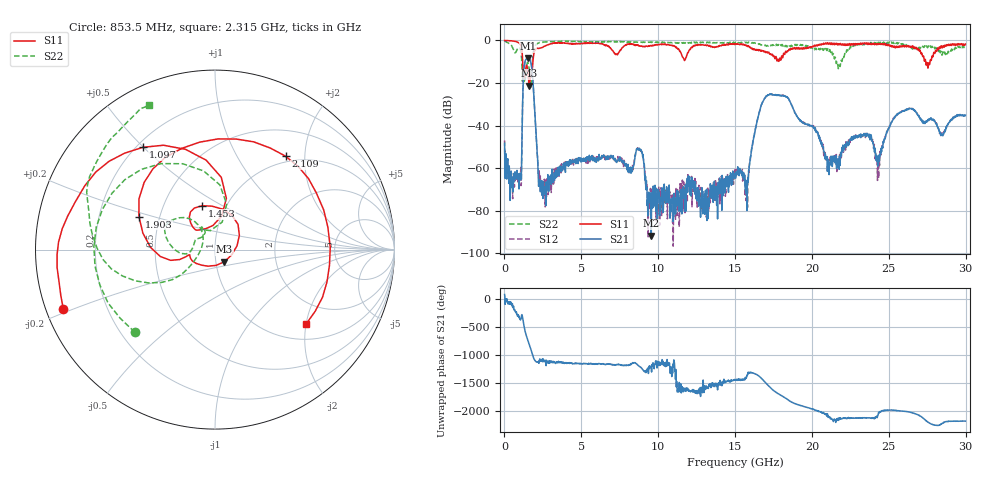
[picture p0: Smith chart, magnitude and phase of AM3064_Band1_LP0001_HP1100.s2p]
# Hz S DB R 50.0
!freq dBS11 angS11 dBS21 angS21 dBS12 angS12 dBS22 angS22
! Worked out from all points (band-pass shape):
!   1600 points, 10 MHz to 29.98 GHz, reference 50 ohm
!   highest |S21| = -8.39 dB at 1.528 GHz (marker M1); lowest = -91.7 dB at 9.551 GHz (marker M2)
!   |S21| within 3 dB of the highest: 1.301 GHz to 1.745 GHz (443.5 MHz wide, 29.1 % of centre)
!   lowest |S11| = -21.4 dB at 1.603 GHz (marker M3), VSWR 1.19, Z = 55 - j7.47 ohm
!   |S11| at or under -10 dB: 1.186 GHz to 1.85 GHz (664 MHz wide, 43.7 % of centre); 27.4 GHz to 27.68 GHz (283.1 MHz wide, 1.03 % of centre)
!   |S22| runs from -22.4 to -0.2 dB; largest |S21 - S12| = 0.0049
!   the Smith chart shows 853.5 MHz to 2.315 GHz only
!   S11 on the Smith chart (normalised r, x): 853.5 MHz: 0.05, -0.19; 1.097 GHz: 0.22, +0.50; 1.453 GHz: 0.77, +0.40; 1.903 GHz: 0.38, +0.18; 2.109 GHz: 0.90, +1.63; 2.315 GHz: 1.36, -2.00
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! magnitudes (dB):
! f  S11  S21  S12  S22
! 10 MHz  -0.1  -48.4  -46.9  -0.2
! 853.5 MHz  -0.8  -64.2  -63.4  -3.9
! 1.097 GHz  -3.1  -65.2  -67.3  -7.1
! 1.453 GHz  -11.9  -8.6  -8.5  -11.7
! 1.528 GHz  -14.4  -8.4  -8.4  -10.5
! 1.603 GHz  -21.4  -8.6  -8.6  -13.0
! 1.903 GHz  -6.7  -25.1  -25.1  -4.6
! 2.109 GHz  -3.7  -50.1  -51.2  -1.7
! 2.315 GHz  -3.7  -67.6  -67.2  -1.1
! 5.015 GHz  -1.4  -56.3  -56.5  -0.8
! 8.782 GHz  -2.7  -51.5  -51.6  -1.0
! 9.551 GHz  -2.6  -91.7  -77.2  -1.0
! 10 GHz  -2.0  -73.8  -77.8  -0.9
! 15 GHz  -1.9  -64.3  -61.9  -1.3
! 15.75 GHz  -2.4  -69.0  -70.0  -0.9
! 17.14 GHz  -5.8  -25.5  -25.6  -2.6
! 19.99 GHz  -3.3  -40.4  -40.2  -3.4
! 21.15 GHz  -1.5  -57.8  -57.9  -4.3
! 23.46 GHz  -1.7  -44.4  -44.3  -1.4
! 24.26 GHz  -1.6  -55.7  -65.8  -1.4
! 25 GHz  -1.9  -41.2  -41.1  -1.1
! 29.98 GHz  -1.7  -35.2  -35.3  -3.1
